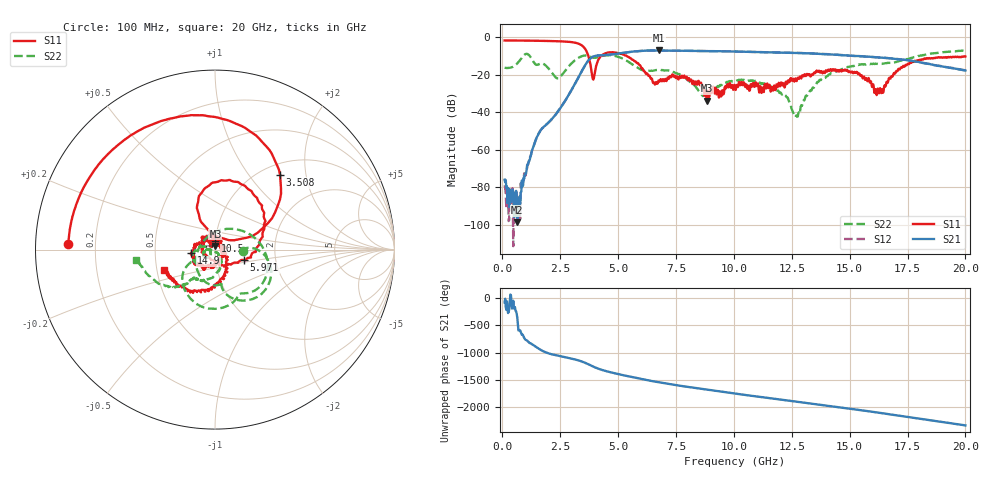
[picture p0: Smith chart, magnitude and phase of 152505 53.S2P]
!  2-Port S-parameters saved by WinCal
! VAR MeasName=S-Parameters (CALIBRATED_DATA) read from VNA (N5230C)
! VAR MeasDate=4/10/2015 9:33:56 AM
! VAR NAME=152505 53
! VAR FILENAME=152505 53.S2P
! VAR DATE=4/10/2015 9:33:57 AM
! VAR PHYS_PORTS=1,2
# Hz S DB R 50
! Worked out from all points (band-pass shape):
!   801 points, 100 MHz to 20 GHz, reference 50 ohm
!   highest |S21| = -7.09 dB at 6.766 GHz (marker M1); lowest = -98.8 dB at 647.2 MHz (marker M2)
!   |S21| within 3 dB of the highest: 3.982 GHz to 15.43 GHz (11.45 GHz wide, 118 % of centre)
!   lowest |S11| = -33.9 dB at 8.831 GHz (marker M3), VSWR 1.04, Z = 50.2 + j2 ohm
!   |S11| at or under -10 dB: 3.716 GHz to 4.272 GHz (556.6 MHz wide, 13.9 % of centre); 5.371 GHz to end of sweep
!   |S22| runs from -42.5 to -7.0 dB; largest |S21 - S12| = 0.0061
!   S11 on the Smith chart (normalised r, x): 100 MHz: 0.10, +0.02; 3.508 GHz: 1.20, +1.44; 5.971 GHz: 1.37, -0.16; 10.5 GHz: 1.00, +0.09; 14.9 GHz: 0.77, -0.03; 20 GHz: 0.55, -0.14
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1e8  -1.75 177.6  -76.07 -83.2  -78.99 -106.4  -16.27 -2.2
6.4725e8  -1.78 164.6  -98.78 2.9  -87.16 23.7  -14.00 2.8
1.567625e9  -1.92 141.4  -51.47 154.8  -51.50 155.1  -14.50 -78.1
2.413375e9  -2.17 115.5  -39.50 22.9  -39.49 22.6  -22.00 132.3
3.43325e9  -4.37 57.0  -18.10 -81.7  -18.13 -81.6  -10.16 -19.1
3.507875e9  -5.15 49.0  -16.45 -93.6  -16.47 -93.6  -9.88 -27.1
3.93075e9  -22.65 76.2  -10.32 -175.9  -10.35 -175.9  -10.92 -59.1
4.5775e9  -8.23 83.0  -9.38 91.5  -9.44 91.7  -9.63 -91.2
5.9705e9  -15.34 -19.6  -7.35 -39.4  -7.33 -39.1  -17.22 -151.5
6.741625e9  -23.19 -158.1  -7.10 -100.9  -7.09 -101.1  -17.40 -151.3
6.7665e9  -23.16 -156.8  -7.09 -102.6  -7.11 -102.8  -17.41 -151.6
7.861e9  -20.47 102.7  -7.30 -177.5  -7.27 -177.3  -21.26 170.2
8.831125e9  -33.93 83.1  -7.39 122.3  -7.44 122.3  -30.72 -155.6
1.005e10  -26.38 118.9  -7.63 51.2  -7.66 51.2  -23.51 -142.2
1.049775e10  -26.60 89.5  -7.77 26.1  -7.78 26.1  -23.10 -153.8
1.221412e10  -25.94 -64.1  -8.24 -69.3  -8.21 -69.7  -30.95 177.9
1.266188e10  -22.01 -75.3  -8.40 -94.2  -8.40 -94.1  -42.54 -153.2
1.338325e10  -19.80 -111.3  -8.71 -134.7  -8.67 -134.6  -27.37 -59.1
1.490062e10  -17.50 -171.6  -9.75 140.3  -9.77 139.5  -15.97 -96.3
1.616925e10  -30.88 63.8  -10.76 67.3  -10.78 67.7  -14.27 -123.1
1.669162e10  -22.04 -33.9  -11.21 36.3  -11.24 36.2  -13.72 -126.6
2e10  -10.29 -157.9  -17.78 -171.4  -17.78 -171.0  -7.02 -172.8
